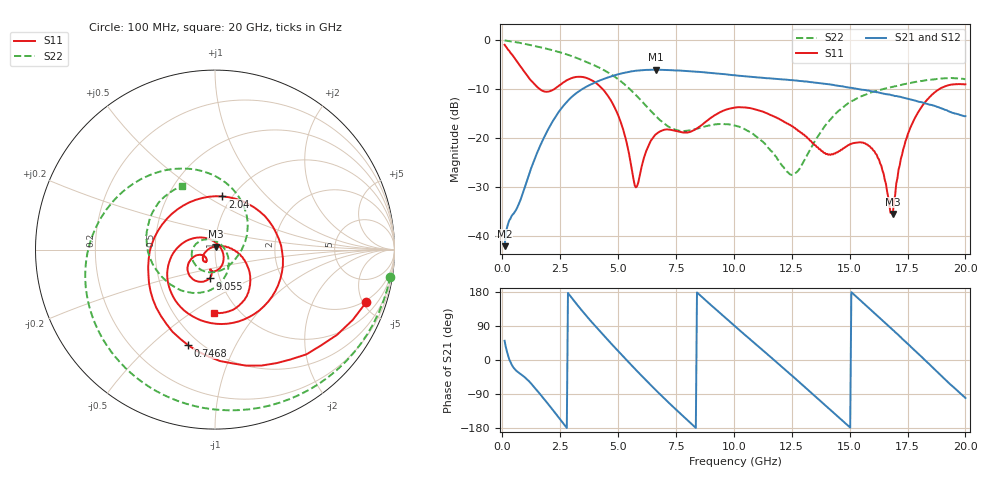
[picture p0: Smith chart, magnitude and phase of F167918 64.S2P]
!  2-Port S-parameters saved by WinCal
! VAR MeasName=S-Parameters (CALIBRATED_DATA) read from VNA (N5242A)
! VAR MeasDate=2016-11-22 10:28:02
! VAR NAME=F167918 64
! VAR FILENAME=F167918 64.S2P
! VAR DATE=2016-11-22 10:28:02
! VAR PHYS_PORTS=1,2
# Hz S DB R 50
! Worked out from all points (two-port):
!   401 points, 100 MHz to 20 GHz, reference 50 ohm
!   highest |S21| = -6.06 dB at 6.617 GHz (marker M1); lowest = -42.1 dB at 100 MHz (marker M2)
!   |S21| within 3 dB of the highest: 3.83 GHz to 14.12 GHz (10.29 GHz wide, 115 % of centre)
!   lowest |S11| = -35.5 dB at 16.87 GHz (marker M3), VSWR 1.03, Z = 50.3 + j1.66 ohm
!   |S11| at or under -10 dB: 1.611 GHz to 2.254 GHz (643.6 MHz wide, 33.3 % of centre); 4.331 GHz to 18.88 GHz (14.55 GHz wide, 125 % of centre)
!   |S22| runs from -27.5 to -0.1 dB; largest |S21 - S12| = 0.005
!   S11 on the Smith chart (normalised r, x): 100 MHz: 1.86, -5.34; 746.8 MHz: 0.43, -0.67; 2.04 GHz: 0.90, +0.59; 9.055 GHz: 0.89, -0.30; 20 GHz: 0.77, -0.62
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1e8  -0.98 -19.0  -42.08 50.7  -42.15 51.7  -0.10 -8.8
7.4675e8  -5.13 -105.6  -33.11 -35.0  -33.11 -34.4  -0.58 -59.8
1.34375e9  -8.77 -178.3  -24.93 -69.3  -24.91 -69.1  -1.17 -100.7
2.04025e9  -10.48 82.1  -17.73 -120.9  -17.72 -120.8  -1.93 -140.9
2.73675e9  -8.36 -7.5  -12.92 -175.3  -12.92 -175.0  -2.86 -175.6
3.43325e9  -7.53 -76.4  -10.08 130.8  -10.03 131.1  -4.08 153.7
4.82625e9  -13.53 177.6  -7.24 35.2  -7.22 34.9  -7.41 94.5
5.7715e9  -30.08 44.1  -6.27 -26.1  -6.28 -26.2  -11.26 51.7
6.61725e9  -19.29 -76.0  -6.06 -78.7  -6.08 -78.7  -15.48 12.3
6.7665e9  -18.80 -83.1  -6.07 -87.7  -6.08 -87.7  -16.17 4.6
7.9605e9  -18.90 -102.4  -6.33 -156.7  -6.32 -156.8  -18.54 -62.1
9.055e9  -15.73 -100.8  -6.74 142.6  -6.72 142.5  -17.36 -121.1
1.005e10  -13.78 -121.4  -7.19 88.9  -7.18 89.0  -17.49 -165.8
1.169175e10  -15.54 -152.0  -7.88 2.4  -7.85 2.1  -23.09 124.3
1.25375e10  -17.63 -160.6  -8.22 -42.7  -8.22 -43.0  -27.51 50.6
1.338325e10  -20.98 -161.3  -8.61 -88.7  -8.59 -88.7  -21.61 -28.7
1.467675e10  -22.35 -127.2  -9.45 -159.3  -9.45 -159.5  -13.91 -86.5
1.587075e10  -21.69 -146.3  -10.40 134.8  -10.43 135.0  -10.82 -126.2
1.67165e10  -33.68 140.0  -11.13 87.9  -11.21 88.2  -9.74 -149.1
1.686575e10  -35.53 79.6  -11.29 79.4  -11.30 79.9  -9.55 -153.0
1.796025e10  -14.74 -22.3  -12.57 16.7  -12.48 17.3  -8.45 179.0
2e10  -9.03 -90.8  -15.55 -100.2  -15.39 -100.4  -8.01 117.7
